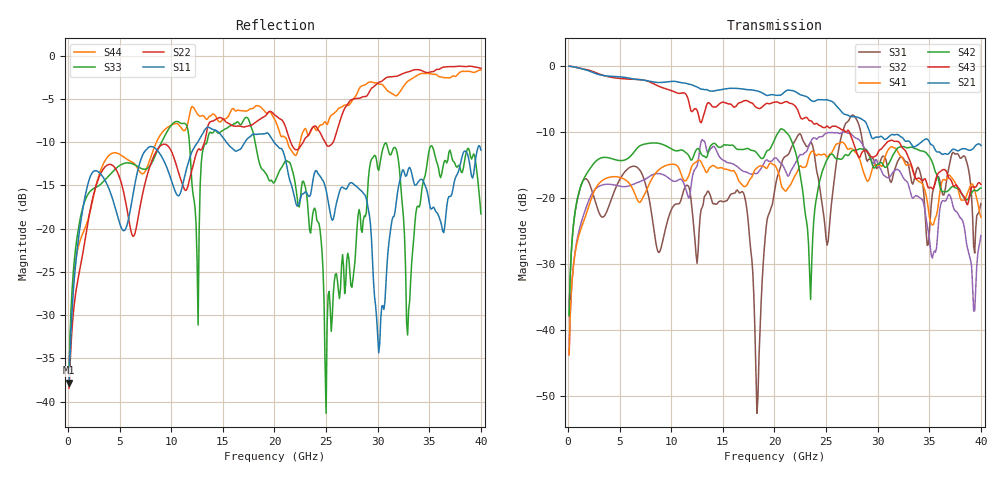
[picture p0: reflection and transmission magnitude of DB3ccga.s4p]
! ADC12DJ3200QML-SP
! 196-pin NWE package
! CCGA Ceramic Package with columns (ceramic column grid array)
! Texas Instruments 4/21/2021
! Single-ended  S-parameters
! PORT#  PORT_NAME  NET_NAME
! PORT1:  DAxN.DIEBUMP DAxN
! PORT2:  DAxN.BGA  DAxN
! PORT3:  DAxP.DIEBUMP DAxP
! PORT4:  DAxP.BGA  DAxP
! Touchstone Ver. 1.0
! Number of ports is 4
# Hz	S	MA	R	50.000000
! SCATTERING PARAMETERS  :
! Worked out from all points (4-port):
!   400 points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, 100 MHz to 40 GHz, reference 50 ohm
!   strongest paths, dB at 100 MHz, 10.1 GHz, 20.1 GHz, 30.1 GHz, 40 GHz:
!     S21: -0.1, -2.4, -4.5, -10.8, -12.1
!     S43: -0.1, -3.8, -5.5, -12.9, -18.0
!     S42: -37.8, -12.7, -10.9, -14.9, -18.5
!     S41: -43.7, -14.9, -15.2, -15.0, -22.9
!     S32: -43.7, -17.4, -14.0, -15.2, -25.7
!     S31: -37.8, -21.5, -18.1, -15.0, -20.9
!   lowest |S11| = -37.8 dB at 100 MHz (marker M1), VSWR 1.03, Z = 51.1 + j0.708 ohm
!   |S11| at or under -10 dB: start of sweep to 12.57 GHz; 15.34 GHz to 17.14 GHz (1.804 GHz wide, 11.1 % of centre); 19.96 GHz to end of sweep
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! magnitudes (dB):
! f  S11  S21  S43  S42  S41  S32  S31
! 100 MHz  -37.8  -0.1  -0.1  -37.8  -43.7  -43.7  -37.8
! 13 GHz  -9.1  -3.6  -8.2  -13.6  -15.0  -11.2  -21.4
! 17.1 GHz  -10.1  -3.6  -5.3  -12.6  -18.3  -16.0  -19.8
! 18.3 GHz  -9.1  -3.8  -6.4  -13.2  -15.5  -16.3  -52.6
! 22.4 GHz  -17.0  -4.3  -7.3  -15.7  -15.4  -13.6  -10.3
! 25 GHz  -15.5  -5.2  -9.3  -14.5  -13.7  -10.2  -26.2
! 40 GHz  -10.9  -12.1  -18.0  -18.5  -22.9  -25.7  -20.9
